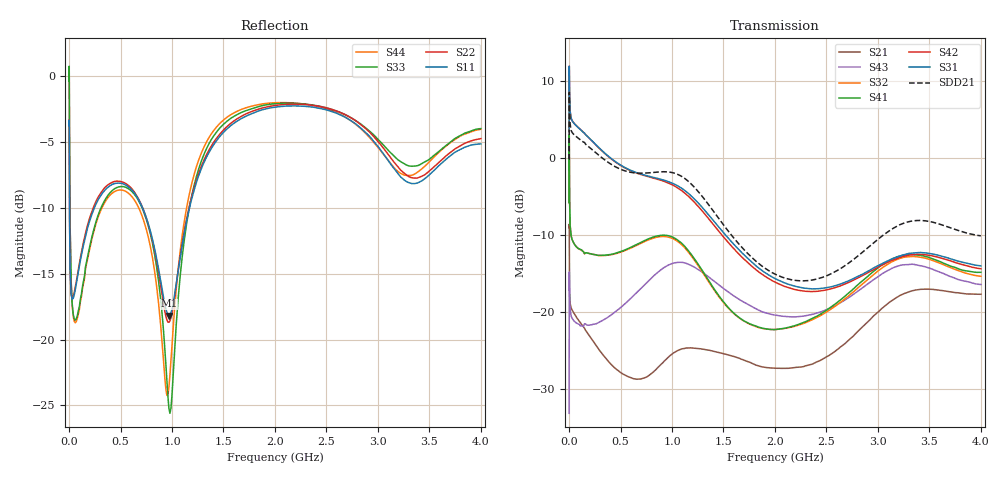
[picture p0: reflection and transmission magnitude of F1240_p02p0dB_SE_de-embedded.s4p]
! Integrated Device Technology
! Corporate Headquarters
! 6024 Silver Creek Valley Road
! San Jose, CA 95138  USA
! Phone:  1-408-284-8200
! Toll Free:  1-800-223-1366
! Webpage:  http://www.idt.com/
! Timing and RF Division
! 515 Groton Road, Suite 102
! Westford, MA 01886-6024
! Device:  F1240
! Description: Dual Intermediate Frequency Digital Variable Gain Amplifier
! Frequency:  10.0 -  500.00 MHz
! Package:  5x5 mm QFN Plastic Package: 32 pin
! Ports:  8 RF, 20 DC
!  Pin  1  = GA3 / Data  Pin 17  = RF OUT_B+
!  Pin  2  = GA4 / CLK  Pin 18  = RF OUT_B-
!  Pin  3  = GA5  Pin 19  = STBY_B
!  Pin  4  = VMODE  Pin 20  = Ground
!  Pin  5  = No Connect  Pin 21  = Ground
!  Pin  6  = GB5  Pin 22  = STB_A
!  Pin  7  = GB4  Pin 23  = RF OUT_A-  = Port 4
!  Pin  8  = GB3  Pin 24  = RF OUT_A+  = Port 3
!  Pin  9  = GB2  Pin 25  = GA0
!  Pin 10  = GB1  Pin 26  = ISET_A
!  Pin 11  = RF IN_B+  Pin 27  = VCC
!  Pin 12  = RF IN_B-  Pin 28  = Ground
!  Pin 13  = Ground  Pin 29  = RF IN_A-  = Port 2
!  Pin 14  = VCC  Pin 30  = RF IN_A+  = Port 1
!  Pin 15  = ISET_B  Pin 31  = GA1
!  Pin 16  = GB0  Pin 32  = GA2 / CSb
! Gain  = +19.5 dB
! State  = 1
! Voltage  = +5.00 V
! Current  = 85.292 mA (one channel only)
! Temperture  =  +25 C
! Test Date  =  2017-10-18
! Board  =  EB4031
! Data:  The device was measured on a custom evaluation board which has
!  individual transmission lines to the RF pins.  Data was collected
!  using a calibrated network analyzer.  The evaluation board was
!  de-embedded using Automatic Fixture Removal.
!  The reference plane is the edge of the package pin.
!  Only Channel A was measured.
!  This data is in single-ended operation.  If your needs are balanced
!  or differential S-parameters then this file needs to be used a
!  linear simulator.
! File Date:  2017-11-10  MJV
! Note:
!  Integrated Device Technology supplies this data as a sample of measured
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# Hz S dB R 100
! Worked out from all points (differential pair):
!   410 points, 500 kHz to 4 GHz, reference 100 ohm
!   strongest paths, dB at 500 kHz, 930 MHz, 1.96 GHz, 2.98 GHz, 4 GHz:
!     S31: 3.5, -2.9, -15.4, -14.1, -14.0
!     S42: 3.5, -3.1, -15.8, -14.3, -14.4
!     S41: -5.8, -10.0, -22.3, -14.5, -14.9
!     S32: -5.8, -10.2, -22.3, -14.9, -15.4
!     S43: -33.2, -14.2, -20.3, -15.6, -16.4
!     S21: -9.0, -26.4, -27.3, -20.3, -17.7
!   taken as a pair (ports 1,2 in; 3,4 out), SDD21 dB: -0.2, -1.8, -14.8, -10.8, -10.1
!   lowest |S11| = -18.2 dB at 970 MHz (marker M1), VSWR 1.28, Z = 79.4 - j8.24 ohm
!   |S11| at or under -10 dB: 4.427 MHz to 245.9 MHz (241.5 MHz wide, 193 % of centre); 713.8 MHz to 1.17 GHz (456 MHz wide, 48.4 % of centre)
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500000  -3.76 -5.5  -9.04 -5.7  -29.23 81.8  -39.37 79.4
        -9.04 -5.7  -3.76 -5.5  -39.33 78.4  -29.23 82.9
        3.48 -106.3  -5.79 -107.4  -0.39 1.1  -33.21 -51.2
        -5.80 -106.3  3.47 -105.2  -33.22 -51.5  -0.40 3.4
2500000  -5.92 -47.1  -12.54 -47.2  -18.51 28.3  -30.40 1.1
         -12.56 -47.2  -5.89 -47.2  -30.36 0.7  -18.51 28.5
         11.40 -179.7  1.13 159.1  -0.94 -54.1  -14.85 -150.4
         1.09 159.2  11.39 -179.4  -14.83 -150.4  -1.00 -53.7
4500000  -10.12 -55.3  -16.82 -39.1  -18.46 12.0  -33.18 -14.5
         -16.82 -39.2  -10.08 -55.5  -33.16 -14.7  -18.47 12.1
         8.77 163.5  -4.35 140.8  -5.09 -79.0  -17.05 178.4
         -4.39 140.8  8.77 163.6  -17.02 178.3  -5.15 -79.0
1.7e8  -11.82 -113.1  -22.58 -51.7  -20.48 -44.8  -36.31 -15.9
       -22.60 -51.6  -11.59 -114.5  -36.39 -15.5  -20.50 -45.0
       2.94 116.5  -12.34 79.4  -14.10 -131.2  -21.78 108.0
       -12.32 79.4  2.94 115.8  -21.72 107.7  -14.24 -130.7
5.2e8  -8.16 -165.8  -28.12 -96.3  -22.07 -109.9  -32.63 -68.9
       -28.08 -95.3  -8.04 -167.4  -32.77 -66.9  -22.23 -110.3
       -1.05 24.8  -12.14 -46.5  -8.38 -169.4  -19.43 11.9
       -12.07 -47.5  -1.10 23.6  -19.23 11.7  -8.66 -169.9
9.7e8  -18.18 -155.5  -26.09 -130.1  -21.06 152.6  -29.85 -159.0
       -25.84 -133.0  -18.69 -153.8  -29.92 -153.0  -21.58 151.2
       -3.08 -86.3  -10.29 172.9  -25.25 -165.5  -14.16 -104.8
       -10.11 169.6  -3.27 -88.8  -13.89 -105.1  -23.62 -129.8
4e9  -5.14 -140.7  -17.74 103.5  -24.12 -47.4  -25.05 -30.7
     -17.71 103.3  -4.75 -139.2  -25.89 -15.0  -25.86 -40.9
     -14.03 36.6  -15.38 -69.2  -3.98 -134.9  -17.85 67.6
     -14.86 -82.8  -14.40 42.5  -16.45 58.0  -4.03 -144.5
